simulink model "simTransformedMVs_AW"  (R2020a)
settings: Solver=ode23s  StartTime=0.0  StopTime=tsim  RelTol=1e-3
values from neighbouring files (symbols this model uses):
  d0 = [T10;T20]    [runTransformedMVs.m]    (also in runTransformedMVsIS.m; Main.m = [Fh, Tcin, Thin]; Main_OL.m = [Fh, Tcin, Thin]; runTestCalcBlk.m = [Fh, Tcin, Thin])
  Kc = 1/k*tau/(tauC+theta)    [Main.m]    (also in runTransf.m = 1/kM(i)*tau(i)/(tauCM(i)+theta(i)); runTransfOL.m = 1/kM(i)*tau(i)/(tauCM(i)+theta(i)))
  KI = Kp/tauIv    [Main.m]    (also in Main_OL.m = 1; runTransf.m = 1/kS(i)*1/tauCS(i); runTransfOL.m = 1/kS(i)*1/tauCS(i))
  p = [V;A(i);B(i)]    [runTransformedMVs.m]    (also in runTransformedMVsIS.m; Main.m = [N, Fc0, rhoc, rhoh,U,A,cpc,cph]; Main_OL.m = [N, Fc0, rhoc, rhoh,U,A,cpc,cph]; runTestCalcBlk.m = [N, Fc0, rhoc, rhoh,U,A,cpc,cph])
  q0 = 10    [runTransformedMVs.m]    (also in runTransformedMVsIS.m)
  qmin = 0    [runTransformedMVs.m]    (also in runTransformedMVsIS.m = -inf)
  T0 = 35    [runTransformedMVs.m]    (also in runTransformedMVsIS.m; H2P_Turbine_driven.m = param(9); runTD.m = 318; H2P_Boiler_driven.m = param(9))
  tauI = min(tau,4*(tauC+theta))    [Main.m]    (also in runTransf.m = min(tau(i), 4*(tauCM(i)+theta(i))); runTransfOL.m = min(tau(i), 4*(tauCM(i)+theta(i))))
  v10 = q0    (= 10)    [runTransformedMVs.m]    (also in runTransformedMVsIS.m)
  v20 = B(i)^(-1)*(f20-A(i)*T0)    [runTransformedMVs.m]    (also in runTransformedMVsIS.m; runTransfOL.m = v00)
undefined symbols (not defined in the file or in its folder): df, InputTransf, InvInputTransf, qf, qmax, tauT, td, TempMixDAE, Tf, tq, tT

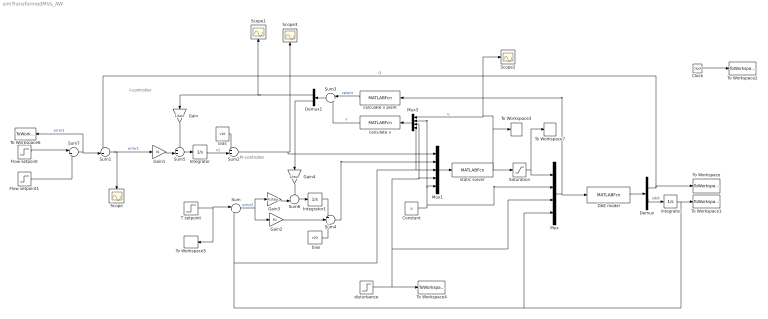
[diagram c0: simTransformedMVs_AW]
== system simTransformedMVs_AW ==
  note: PI-controller
  note: I-controller
  "  bias" : Constant  Value=v20
  " integrator" : Integrator  InitialCondition=T0
  Clock : Clock
  Constant : Constant  Value=p
  DAE model : MATLABFcn  MATLABFcn=TempMixDAE(u(1:2), u(3),u(4:5),u(6))  OutputDimensions=2
  Demux : Demux  Outputs=2
  Demux1 : Demux  Outputs=2
  Flow setpoint : Step  Time=tq  Before=q0  After=qf  SampleTime=0
  Flow setpoint1 : Step  Time=tq*2  After=q0-qf  SampleTime=0
  Gain : Gain  Gain=1/tauT  Multiplication=Matrix(K*u)
  Gain1 : Gain  Gain=KI  Multiplication=Matrix(K*u)
  Gain2 : Gain  Gain=Kc  Multiplication=Matrix(K*u)
  Gain3 : Gain  Gain=Kc/tauI  Multiplication=Matrix(K*u)
  Gain4 : Gain  Gain=1/tauT  Multiplication=Matrix(K*u)
  Integrator : Integrator
  Integrator1 : Integrator
  Mux : Mux
  Mux1 : Mux  Inputs=5
  Mux3 : Mux
  Saturation : Saturate  UpperLimit=qmax  LowerLimit=qmin
  Scope{,1..3} (4 alike) : Scope
  Sum : Sum  Inputs=|+-
  Sum1 : Sum  Inputs=-+|
  Sum2 : Sum  Inputs=++|
  Sum3 : Sum  Inputs=|+-
  Sum4 : Sum  Inputs=+++
  Sum5 : Sum  Inputs=++|
  Sum6 : Sum  Inputs=++|
  Sum7 : Sum  Inputs=|++
  T setpoint : Step  Time=tT  Before=T0  After=Tf  SampleTime=0
  To Workspace : ToWorkspace  VariableName=q  SampleTime=-1
  To Workspace1 : ToWorkspace  VariableName=T  SampleTime=-1
  To Workspace2 : ToWorkspace  VariableName=time  SampleTime=-1
  To Workspace3 : ToWorkspace  VariableName=u  SampleTime=-1
  To Workspace4 : ToWorkspace  VariableName=d  SampleTime=-1
  To Workspace5 : ToWorkspace  VariableName=Ts  SampleTime=-1
  To Workspace6 : ToWorkspace  VariableName=qs  SampleTime=-1
  To Workspace7 : ToWorkspace  VariableName=uplant  SampleTime=-1
  bias : Constant  Value=v10
  calculate v : MATLABFcn  MATLABFcn=InputTransf(u(1:2),u(3),u(4:5),u(6))  OutputDimensions=2
  calculate v plant : MATLABFcn  MATLABFcn=InputTransf(u(1:2),u(3),u(4:5),u(6))  OutputDimensions=2
  disturbance : Step  Time=td  Before=d0  After=df  SampleTime=0
  static solver : MATLABFcn  MATLABFcn=InvInputTransf(u(1:2),u(3),u(4:5),u(6))  OutputDimensions=2
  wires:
  DAE model/1 -> Demux/1
  Demux/1 -> To Workspace/1, Sum1/1  "q"
  " integrator"/1 -> To Workspace1/1, Mux/4, Mux3/4, Mux1/3, Sum/2  "T"
  Mux/1 -> calculate v plant/1, DAE model/1
  Clock/1 -> To Workspace2/1
  Sum/1 -> Gain2/1, Gain3/1  "error2"
  T setpoint/1 -> To Workspace5/1, Sum/1
  Sum1/1 -> Gain1/1, Scope/1  "error1"
  Gain1/1 -> Sum5/2
  bias/1 -> Sum2/1
  Mux1/1 -> static solver/1
  Sum2/1 -> Scope3/1, Mux1/1
  Sum4/1 -> Mux1/2
  Demux/2 -> " integrator"/1  "xdot"
  Integrator/1 -> Sum2/2  "v1"
  Gain3/1 -> Sum6/2
  Integrator1/1 -> Sum4/1
  Constant/1 -> Mux/2, Mux3/2, Mux1/5
  disturbance/1 -> To Workspace4/1, Mux/3, Mux3/3, Mux1/4
  static solver/1 -> To Workspace3/1, Scope2/1, Mux3/1, Saturation/1  "u"
  Saturation/1 -> To Workspace7/1, Mux/1
  Sum5/1 -> Integrator/1
  calculate v plant/1 -> Sum3/1  "vplant"
  calculate v/1 -> Sum3/2  "v"
  Sum3/1 -> Demux1/1
  Demux1/1 -> Scope1/1, Gain/1
  Gain/1 -> Sum5/1
  "  bias"/1 -> Sum4/3
  Gain2/1 -> Sum4/2
  Sum6/1 -> Integrator1/1
  Demux1/2 -> Gain4/1
  Gain4/1 -> Sum6/1
  Mux3/1 -> calculate v/1
  Sum7/1 -> Sum1/2, To Workspace6/1  "error1"
  Flow setpoint1/1 -> Sum7/2
  Flow setpoint/1 -> Sum7/1
